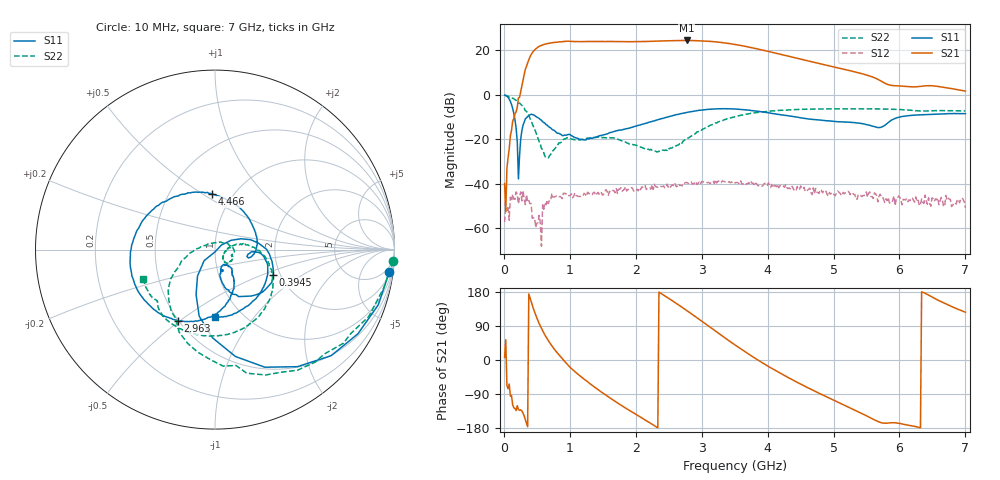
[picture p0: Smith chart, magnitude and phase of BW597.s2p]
!Agilent Technologies,N5244A,MY49441013,A.09.90.07
!Agilent N5244A: A.09.90.07
!Date: Wednesday, May 21, 2014 11:04:21
!Correction: S11(Full 2 Port with power(1,2))
!S21(Full 2 Port with power(1,2))
!S12(Full 2 Port with power(1,2))
!S22(Full 2 Port with power(1,2))
!S2P File: Measurements: S11, S21, S12, S22:
# Hz S  dB  R 50
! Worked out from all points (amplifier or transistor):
!   401 points, 10 MHz to 7 GHz, reference 50 ohm
!   highest |S21| = 24.5 dB at 2.771 GHz (marker M1)
!   |S21| within 3 dB of that: 516.4 MHz to 3.717 GHz (3.2 GHz wide, 151 % of centre)
!   unconditionally stable (mu >= 1): start of sweep to end of sweep
!   at 1.163 GHz: K = 6.10, MAG = 24.0 dB, |S12| = -45.8 dB
!   at 3.505 GHz: K = 2.56, MAG = 24.3 dB, |S12| = -39.7 dB
!   at 7 GHz: K = 100.94, MAG = 3.2 dB, |S12| = -50.9 dB
!   S11 on the Smith chart (normalised r, x): 10 MHz: 3, -15; 394.4 MHz: 1.84, -0.59; 2.963 GHz: 0.49, -0.49; 4.466 GHz: 0.80, +0.55; 7 GHz: 0.75, -0.66
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1e7  -0.18 -7.2  -40.05 7.0  -57.33 -165.1  -0.05 -3.8
2.5465e8  -19.76 30.1  1.47 -131.5  -43.74 26.8  -4.24 -92.3
3.9445e8  -9.04 -23.4  17.01 164.5  -49.04 -67.9  -10.56 -146.4
5.16775e8  -10.32 -58.9  21.49 103.5  -57.64 69.1  -19.51 177.8
6.21625e8  -12.79 -73.9  22.80 65.8  -48.52 45.7  -27.71 123.4
7.4395e8  -15.83 -78.5  23.49 33.3  -46.10 38.2  -25.17 46.1
8.66275e8  -17.85 -75.8  23.87 6.8  -46.05 17.6  -21.42 12.6
1.180825e9  -20.12 -65.4  23.94 -45.7  -45.45 -3.5  -20.11 -20.5
1.425475e9  -18.76 -51.2  24.02 -78.1  -43.95 -4.0  -19.11 -31.9
1.670125e9  -16.54 -50.3  23.99 -107.2  -43.17 -17.7  -19.46 -45.0
2.019625e9  -13.89 -58.0  23.95 -145.3  -42.43 -34.4  -22.96 -49.7
2.35165e9  -11.09 -72.1  24.22 179.1  -41.44 -49.5  -25.44 -25.2
2.77105e9  -8.01 -100.6  24.48 130.7  -39.50 -69.1  -19.73 12.7
2.963275e9  -6.97 -117.5  24.34 107.2  -39.36 -75.9  -16.44 10.3
3.207925e9  -6.38 -140.7  23.86 76.6  -38.31 -97.9  -12.61 1.9
3.505e9  -6.39 -170.9  22.67 39.8  -39.67 -123.0  -9.85 -16.7
3.9943e9  -8.00 140.2  19.66 -15.2  -40.79 -145.9  -7.51 -47.2
4.466125e9  -10.18 92.7  16.34 -60.4  -42.69 -174.3  -6.61 -71.1
4.675825e9  -11.05 70.5  14.82 -78.8  -45.00 170.5  -6.45 -80.7
5.2525e9  -12.37 12.5  10.82 -126.5  -45.00 146.6  -6.30 -103.2
5.84665e9  -12.06 -4.2  4.43 -166.0  -48.71 115.1  -6.46 -124.3
7e9  -8.50 -89.8  1.67 126.1  -50.89 70.5  -7.28 -157.4
